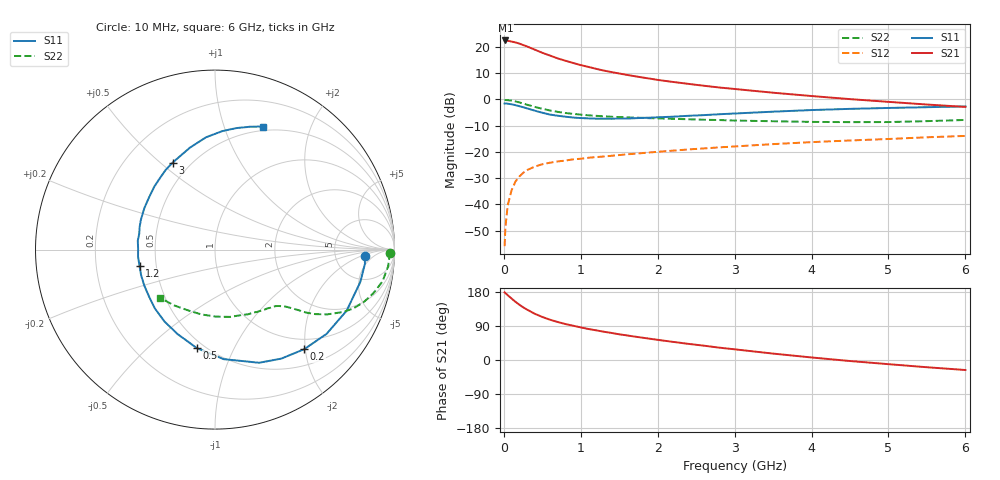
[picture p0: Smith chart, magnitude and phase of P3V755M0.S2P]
! SIEMENS Small Signal Semiconductors
! BFP181
! Si NPN RF Bipolar Junction Transistor in SOT143
! VCE = 0.75 V  IC = 5 mA
! Common Emitter S-Parameters:  March  1996
# GHz  S  MA  R  50
!  f  S11  S21  S12  S22
! GHz  MAG  ANG  MAG  ANG  MAG  ANG  MAG  ANG
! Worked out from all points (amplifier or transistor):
!   36 points, 10 MHz to 6 GHz, reference 50 ohm
!   highest |S21| = 22.5 dB at 20 MHz (marker M1)
!   |S21| within 3 dB of that: start of sweep to 360.6 MHz
!   unconditionally stable (mu >= 1): 1.193 GHz to end of sweep
!   at 250 MHz: K = 0.27, MSG = 24.4 dB, |S12| = -28.0 dB
!   at 1.4 GHz: K = 1.10, MAG = 14.0 dB, |S12| = -21.5 dB
!   at 6 GHz: K = 1.22, MAG = 2.7 dB, |S12| = -13.9 dB
!   S11 on the Smith chart (normalised r, x): 10 MHz: 10, -3; 200 MHz: 0.79, -1.98; 500 MHz: 0.45, -0.72; 1.2 GHz: 0.40, -0.09; 3 GHz: 0.40, +0.55; 6 GHz: 0.45, +1.36
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0.01  0.8345 -2.6  13.17 178.4  0.0016 84.7  0.9771 -1.0
0.02  0.8393 -5.4  13.3 176.8  0.0036 90.0  0.9733 -2.1
0.05  0.8294 -12.6  13.13 171.1  0.0096 85.0  0.9689 -5.5
0.1  0.8086 -24.9  12.67 162.3  0.0185 75.9  0.9504 -10.7
0.15  0.779 -37.1  12.21 153.7  0.0271 69.8  0.9152 -15.4
0.2  0.7447 -48.2  11.62 146.2  0.0338 64.7  0.8783 -19.5
0.25  0.7109 -58.7  10.89 139.1  0.0398 60.1  0.8369 -23.1
0.3  0.6767 -68.7  10.24 133.2  0.0449 56.1  0.7953 -25.9
0.4  0.6122 -85.5  8.913 122.2  0.0524 50.0  0.7221 -30.0
0.5  0.5577 -100.5  7.737 113.6  0.0583 45.1  0.6636 -32.8
0.6  0.5148 -113.9  6.856 106.3  0.0623 42.5  0.6159 -34.7
0.7  0.4897 -125.0  6.047 100.3  0.0658 40.3  0.5795 -35.8
0.9  0.4518 -144.2  4.959 90.5  0.0722 37.9  0.5308 -37.7
1.1  0.4355 -161.1  4.163 81.8  0.0774 36.8  0.4985 -39.4
1.2  0.4303 -167.7  3.83 78.3  0.0797 36.1  0.4869 -40.4
1.7  0.4388 163.0  2.773 61.8  0.0922 35.1  0.4502 -45.6
2.2  0.469 141.5  2.153 47.8  0.1059 33.9  0.4268 -52.6
3  0.5393 115.9  1.582 28.2  0.1271 30.4  0.3958 -66.6
3.5  0.5846 103.9  1.343 16.9  0.1408 27.7  0.3842 -77.4
4.5  0.6613 86.5  1.014 -2.7  0.1652 20.9  0.3691 -101.8
5.5  0.7117 74.1  0.8 -19.1  0.1901 14.7  0.386 -126.6
6  0.7355 68.8  0.72 -26.4  0.2017 11.0  0.4064 -138.4
